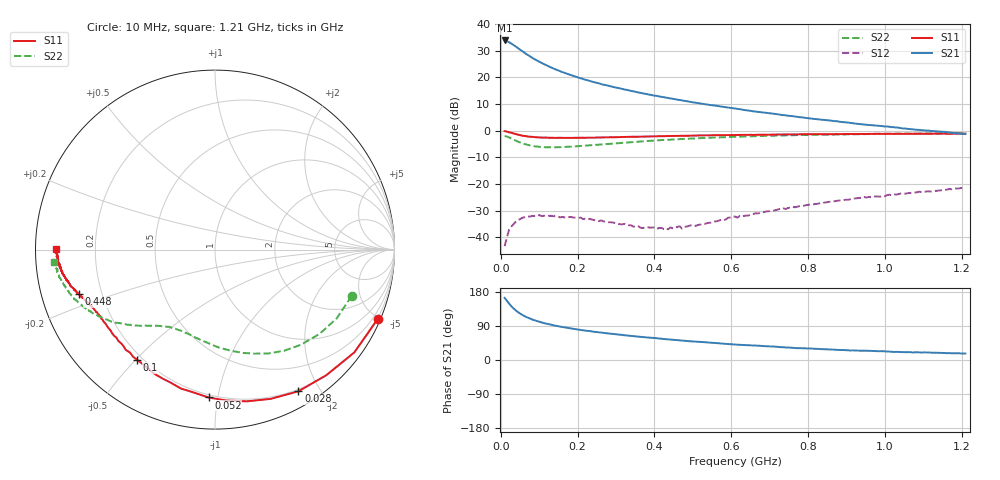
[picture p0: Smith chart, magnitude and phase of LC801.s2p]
!  POLYFET RF DEVICES
!  S PARAMETERS FOR
!  LC801
!  VDS=28, IDQ=200mA
# MHZ S MA R 50
! SCATTERING PARAMETERS :
!  FREQ  S11 MAG  S11 ANG  S21 MAG  S21 ANG  S12 MAG  S12 ANG  S22 MAG  S22 ANG
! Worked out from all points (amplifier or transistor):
!   201 points, 10 MHz to 1.21 GHz, reference 50 ohm
!   highest |S21| = 33.9 dB at 10 MHz (marker M1)
!   |S21| within 3 dB of that: start of sweep to 45.93 MHz
!   unconditionally stable (mu >= 1): 343.9 MHz to 589.2 MHz; 615.3241 MHz to 616.7 MHz
!   at 208 MHz: K = 0.45, MSG = 26.1 dB, |S12| = -32.5 dB
!   at 610 MHz: K = 0.95, MSG = 20.2 dB, |S12| = -32.2 dB
!   at 1.21 GHz: K = 0.59, MSG = 10.1 dB, |S12| = -21.4 dB
!   S11 on the Smith chart (normalised r, x): 10 MHz: 0.19, -4.87; 28 MHz: 0.18, -1.74; 52 MHz: 0.18, -0.94; 100 MHz: 0.18, -0.50; 448 MHz: 0.11, -0.16; 1.21 GHz: 0.06, +0.00
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10  0.985 -23.2  49.37 164.0  0.00687 72.2  0.8034 -18.8
16  0.9647 -36.4  47.7 156.1  0.01007 65.5  0.779 -29.5
22  0.935 -48.5  45.56 148.2  0.01421 61.3  0.7483 -38.9
28  0.916 -59.5  42.87 141.5  0.01613 54.8  0.7142 -47.9
34  0.8877 -69.5  40.24 135.4  0.01807 48.1  0.6825 -55.7
40  0.8637 -78.2  37.45 130.2  0.02013 45.3  0.6498 -63.0
52  0.8247 -92.5  32.57 121.5  0.02238 36.0  0.5966 -74.7
64  0.797 -103.7  28.19 114.8  0.02401 31.9  0.5586 -84.1
70  0.7812 -108.4  26.43 111.9  0.02479 27.9  0.5446 -88.1
82  0.7692 -116.4  23.36 106.9  0.02542 24.5  0.5208 -94.7
100  0.7517 -125.3  19.7 100.9  0.02631 20.5  0.5016 -102.5
118  0.7479 -131.7  16.96 96.1  0.02539 18.0  0.4914 -108.6
142  0.7365 -138.3  14.24 90.7  0.02509 15.9  0.4909 -114.3
178  0.7369 -144.8  11.37 84.0  0.02416 13.0  0.5009 -120.7
214  0.7393 -149.3  9.357 78.5  0.02217 11.4  0.5218 -125.3
292  0.755 -155.2  6.655 68.6  0.01911 17.3  0.5764 -132.9
412  0.7923 -160.7  4.418 56.6  0.0151 39.9  0.6633 -141.6
448  0.8 -161.9  3.97 53.4  0.01485 48.9  0.6881 -143.7
610  0.8331 -166.9  2.608 40.8  0.02465 85.6  0.7722 -153.2
814  0.8589 -172.0  1.676 29.8  0.04201 96.4  0.8406 -162.5
1012  0.8774 -176.2  1.191 22.2  0.06326 98.0  0.8777 -169.5
1210  0.8866 179.8  0.8672 17.2  0.08525 97.1  0.9 -175.6
